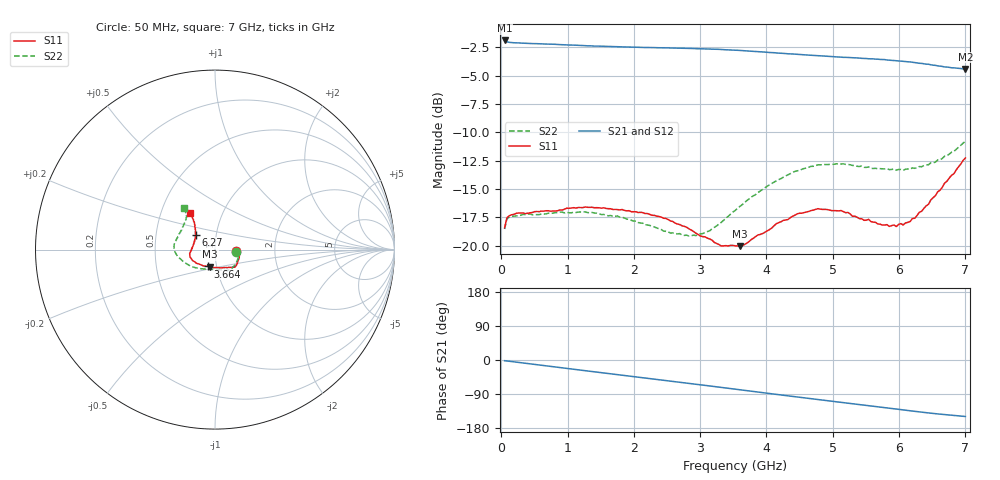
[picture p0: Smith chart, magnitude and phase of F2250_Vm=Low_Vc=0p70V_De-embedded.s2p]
! Integrated Device Technology
! Corporate Headquarters
! 6024 Silver Creek Valley Road
! San Jose, CA 95138  USA
! Phone:  1-408-284-8200
! Toll Free:  1-800-223-1366
! Webpage:  http://www.idt.com/
! Timing and RF Division
! 515 Groton Road, Suite 102
! Westford, MA 01886-6024
! Device:  F2250
! Description: Voltage Variable RF Attenuator
! Frequency:  50.0 -  6000.00 MHz
! Package:  3x3 mm Thin QFN Plastic Package: 16 pin
! Ports:  2 RF, 3 DC
!  Pin  1  = GND
!  Pin  2  = NC
!  Pin  3  = RF1  = Port 1
!  Pin  4  = NC
!  Pin  5  = GND
!  Pin  6  = GND
!  Pin  7  = GND
!  Pin  8  = GND
!  Pin  9  = NC
!  Pin 10  = RF2  = Port 2
!  Pin 11  = NC
!  Pin 12  = GND
!  Pin 13  = GND
!  Pin 14  = VCNTRL
!  Pin 15  = VDD
!  Pin 16  = VMODE
! Vcntrl:  0.700 Volts
! Vmode:  +0.000 Volts
! Vdd:  +3.30  Volts
! Current:  1.149 mA
! Data:  The device was measured on a the F2250 evaluation board which has
!  individual transmission lines to the RF pins.  Data was collected
!  using a calibrated network analyzer.  The evaluation board was
!  de-embedded using a TRL calibration technique.
!  The reference plane is the edge of the package pin.
! Misc:  SN 10
!  Action Tracker AT0258
! Date Measured:  2014-11-26
! Date:  2015-10-15  MJV
! Note:
!  Integrated Device Technology supplies this data as a sample of measured
!  data at the package pin for this product.  Your particular data for this
!  product may vary.
!  Data was taken at 25 degrees C.
!  Integrated Device Technology reserves the right to change this data at anytime.
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# GHz S dB R 50
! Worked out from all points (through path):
!   201 points, 50 MHz to 7 GHz, reference 50 ohm
!   highest |S21| = -1.91 dB at 50 MHz (marker M1); lowest = -4.4 dB at 7 GHz (marker M2)
!   group delay of S21, straight-line fit = 59.8 ps
!   lowest |S11| = -20.0 dB at 3.595 GHz (marker M3), VSWR 1.22, Z = 46.5 - j8.97 ohm
!   |S11| at or under -10 dB: start of sweep to end of sweep
!   |S22| runs from -19.1 to -10.8 dB; largest |S21 - S12| = 0.0011
!   S11 on the Smith chart (normalised r, x): 50 MHz: 1.27, -0.02; 3.664 GHz: 0.91, -0.17; 6.27 GHz: 0.79, +0.13; 7 GHz: 0.71, +0.30
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0.05  -18.41 -4.2  -1.91 -1.9  -1.91 -1.9  -18.52 -5.6
0.08475  -17.53 -4.5  -2.03 -2.5  -2.03 -2.5  -17.63 -5.5
0.22375  -17.14 -8.4  -2.12 -5.5  -2.11 -5.5  -17.37 -10.5
0.77975  -16.93 -25.2  -2.24 -17.8  -2.23 -17.7  -17.12 -32.1
1.2315  -16.64 -36.6  -2.35 -27.5  -2.36 -27.5  -17.03 -48.0
1.75275  -16.81 -43.3  -2.47 -38.4  -2.46 -38.4  -17.37 -59.6
2.37825  -17.42 -47.4  -2.55 -51.7  -2.55 -51.7  -18.50 -72.4
2.93425  -18.89 -61.0  -2.63 -63.8  -2.63 -63.8  -19.10 -97.8
3.14275  -19.40 -72.6  -2.66 -68.4  -2.67 -68.4  -18.68 -111.6
3.3165  -20.01 -84.8  -2.70 -72.3  -2.71 -72.4  -17.94 -122.2
3.525  -20.00 -100.7  -2.77 -77.0  -2.76 -77.0  -16.91 -134.0
3.5945  -20.03 -106.2  -2.79 -78.6  -2.79 -78.6  -16.55 -137.3
3.664  -19.91 -112.2  -2.81 -80.1  -2.80 -80.1  -16.22 -140.6
4.1505  -18.04 -141.4  -3.01 -90.8  -3.01 -90.8  -14.26 -161.8
4.7065  -16.86 -160.9  -3.22 -102.8  -3.23 -102.8  -12.99 -177.2
5.1235  -16.90 -171.0  -3.38 -111.7  -3.38 -111.8  -12.80 173.3
5.471  -17.76 178.5  -3.49 -119.1  -3.49 -119.1  -13.09 165.6
5.85325  -18.29 164.1  -3.64 -127.2  -3.64 -127.2  -13.29 155.7
6.06175  -18.17 154.1  -3.74 -131.7  -3.74 -131.7  -13.35 149.5
6.27025  -17.34 143.1  -3.88 -136.2  -3.88 -136.2  -13.12 142.8
6.61775  -15.10 129.2  -4.17 -142.9  -4.18 -142.9  -12.42 131.3
7  -12.26 124.1  -4.42 -149.1  -4.43 -149.1  -10.80 126.8
